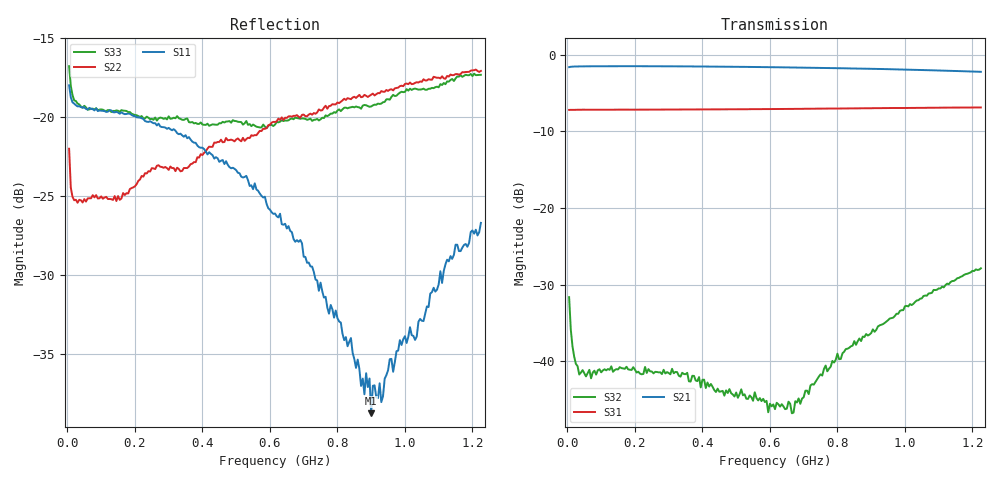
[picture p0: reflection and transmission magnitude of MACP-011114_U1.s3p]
!Agilent Technologies,E5071C,MY46110647,A.11.31
!Date: Tue Jan 09 14:58:34 2024 DD
!Data & Calibration Information:
!MACP-011114 soldered onto PT-0030145 with F connectors, calibration PCB PT-0003653. Port1 (pin1) Port2 (pin6) Port3 (pin3)
!Freq	S11:SOLT3(ON)	S12:SOLT3(ON)	S13:SOLT3(ON)
!	S21:SOLT3(ON)	S22:SOLT3(ON)	S23:SOLT3(ON)
!	S31:SOLT3(ON)	S32:SOLT3(ON)	S33:SOLT3(ON)
!PortZ  Port1:75+j0  Port2:75+j0  Port3:75+j0
!Above PortZ is port z conversion or system Z0 setting when saving the data.
!When reading, reference impedance value at option line is always used.
# Hz S MA R 75
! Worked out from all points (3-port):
!   245 points, 5 MHz to 1.225 GHz, reference 75 ohm
!   strongest paths, dB at 5 MHz, 310 MHz, 615 MHz, 920 MHz, 1.225 GHz:
!     S21: -1.6, -1.5, -1.6, -1.8, -2.2
!     S31: -7.2, -7.1, -7.1, -6.9, -6.9
!     S32: -31.6, -41.0, -46.3, -35.5, -27.9
!   lowest |S11| = -38.8 dB at 900 MHz (marker M1), VSWR 1.02, Z = 76.3 + j1.11 ohm
!   |S11| at or under -10 dB: start of sweep to end of sweep
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5000000  0.1263 159.5  0.8327 2.8  0.4362 -178.7
         0.8323 2.9  0.07948 66.0  0.02486 96.1
         0.4375 -179.0  0.0262 92.6  0.1453 152.9
2e7  0.1105 171.9  0.8402 0.0  0.4383 178.7
     0.84 0.1  0.05457 21.1  0.01033 57.7
     0.4382 178.7  0.01073 61.0  0.1132 166.4
3.5e7  0.1084 173.7  0.8417 -1.0  0.4387 177.1
       0.8412 -1.0  0.05475 10.0  0.009005 41.8
       0.4386 177.1  0.008191 42.5  0.1099 169.2
3.2e8  0.09072 161.2  0.8422 -15.0  0.4398 150.2
       0.8421 -14.9  0.0675 -31.2  0.008232 7.4
       0.4396 150.2  0.008513 16.2  0.09932 143.1
6.15e8  0.04952 134.9  0.8297 -29.2  0.4437 122.8
        0.8309 -29.0  0.09669 -47.6  0.003448 61.7
        0.443 123.0  0.004865 58.1  0.09481 104.3
6.7e8  0.04108 125.4  0.8267 -31.8  0.4444 117.7
       0.828 -31.7  0.1011 -45.9  0.004161 82.9
       0.4442 117.9  0.004623 81.0  0.0986 98.1
7.2e8  0.03368 120.9  0.8233 -34.2  0.4453 113.1
       0.825 -34.1  0.1027 -49.5  0.007093 94.6
       0.4457 113.2  0.006944 82.3  0.09903 92.6
8.95e8  0.01485 47.0  0.8098 -42.8  0.4492 96.8
        0.8117 -42.7  0.117 -51.9  0.01609 107.8
        0.449 97.0  0.01493 100.6  0.108 69.4
9e8  0.01151 39.4  0.8096 -43.1  0.4493 96.3
     0.8114 -43.0  0.1179 -52.4  0.01659 106.4
     0.4491 96.5  0.01527 100.7  0.1082 68.9
1.225e9  0.04625 -60.6  0.7738 -59.6  0.4546 65.4
         0.7758 -59.5  0.1404 -63.0  0.04075 84.2
         0.4538 65.7  0.04043 82.1  0.1364 36.8
